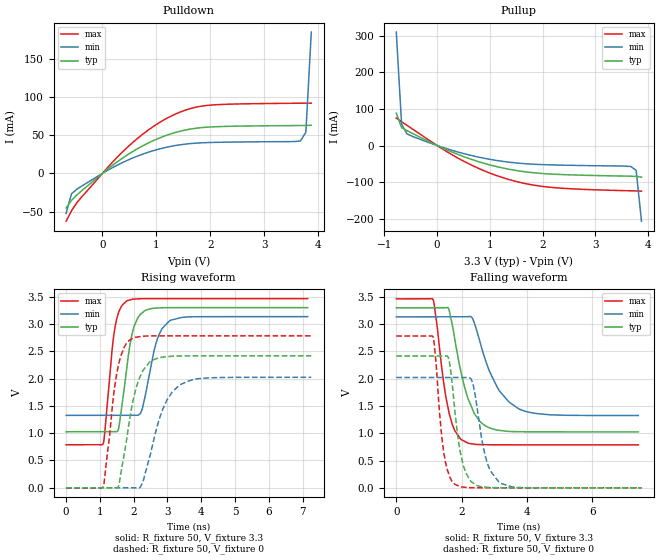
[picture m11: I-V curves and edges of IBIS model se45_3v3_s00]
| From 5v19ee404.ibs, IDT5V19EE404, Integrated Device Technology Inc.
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[Model]   se45_3v3_s00
Model_type   Output
Polarity   Non-Inverting
|   typ   min   max
C_comp   2pF   1.5pF   2.5pF
Vmeas = 1.65V
Rref = 50
Cref = 0
Vref = 1.65V
|   typ   min   max
[Voltage range]   3.3V   3.135V   3.465V
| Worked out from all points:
|   slope of the pulldown table from 0 to 0.495 V, typ, clamps not added: 19.3 ohm
|   slope of the pullup table from 0 to 0.495 V, typ, clamps not added: 16.5 ohm
|   rising waveform, R_fixture 50, V_fixture 3.3: 20-80 % time 317ps typ, 388ps min, 255ps max; typ from 1.03 V to 3.3 V
|   falling waveform, R_fixture 50, V_fixture 3.3: 20-80 % time 546ps typ, 767ps min, 379ps max; typ from 3.3 V to 1.03 V
|   rising waveform, R_fixture 50, V_fixture 0: 20-80 % time 444ps typ, 594ps min, 330ps max; typ from 0 V to 2.42 V
|   falling waveform, R_fixture 50, V_fixture 0: 20-80 % time 314ps typ, 381ps min, 254ps max; typ from 2.42 V to 0 V
[Pulldown]
|Voltage   I (typ)   I (min)   I (max)
|Note, modeling breaks down at 250mA and above.  This is well beyond the functional   |
|operating range of the device.  Should this scenario occur, catastrophic failure and   |
|possible damage to the device and/or board is of higher concern than the I-V curve   |
|behavior.  The IBIS checker will flag currents in excess of 10A with warnings.  Lines   |
|with currents in excess of 0.35 A have been commented out.  The points still remain|
|available to the user if the user desires to use them.   |
|-3.30000e+00   -6.87686e+01   -5.43171e+01   -9.32008e+01
|-3.19898e+00   -6.58203e+01   -5.20452e+01   -8.91014e+01
|-3.09796e+00   -6.28735e+01   -4.97746e+01   -8.50038e+01
|-2.99694e+00   -5.99283e+01   -4.75054e+01   -8.09081e+01
|-2.89592e+00   -5.69850e+01   -4.52379e+01   -7.68145e+01
|-2.79490e+00   -5.40436e+01   -4.29721e+01   -7.27232e+01
|-2.69388e+00   -5.11045e+01   -4.07082e+01   -6.86345e+01
|-2.59286e+00   -4.81679e+01   -3.84464e+01   -6.45487e+01
|-2.49184e+00   -4.52341e+01   -3.61871e+01   -6.04662e+01
|-2.39082e+00   -4.23034e+01   -3.39304e+01   -5.63874e+01
|-2.28980e+00   -3.93763e+01   -3.16768e+01   -5.23129e+01
|-2.18878e+00   -3.64533e+01   -2.94267e+01   -4.82433e+01
|-2.08776e+00   -3.35351e+01   -2.71807e+01   -4.41794e+01
|-1.98673e+00   -3.06226e+01   -2.49393e+01   -4.01225e+01
|-1.88571e+00   -2.77168e+01   -2.27035e+01   -3.60739e+01
|-1.78469e+00   -2.48192e+01   -2.04743e+01   -3.20355e+01
|-1.68367e+00   -2.19317e+01   -1.82533e+01   -2.80101e+01
|-1.58265e+00   -1.90571e+01   -1.60423e+01   -2.40013e+01
|-1.48163e+00   -1.61992e+01   -1.38443e+01   -2.00151e+01
|-1.38061e+00   -1.33643e+01   -1.16633e+01   -1.60610e+01
|-1.27959e+00   -1.05622e+01   -9.50583e+00   -1.21557e+01
|-1.17857e+00   -7.81131e+00   -7.38261e+00   -8.33341e+00
|-1.07755e+00   -5.14939e+00   -5.31366e+00   -4.68044e+00
|-9.76531e-01   -2.67462e+00   -3.34162e+00   -1.51483e+00
|-8.75510e-01   -7.31794e-01   -1.57851e+00   -1.44651e-01
|-7.74490e-01   -8.69816e-02   -3.68375e-01   -7.86452e-02
-673.5mV  -45.24mA   -52.43mA   -62.63mA
-572.4mV  -35.28mA   -26.51mA   -48.86mA
-471.4mV  -27.99mA   -20.59mA   -38.06mA
134.7mV   7.697mA    5.495mA    10.74mA
437.8mV   23.12mA    16.34mA    32.53mA
841.8mV   39.56mA    27.55mA    56.35mA
1.246V    51.27mA    35.11mA    74.04mA
1.65V     58.26mA    39.16mA    85.27mA
1.953V    60.57mA    40.35mA    89.06mA
3.67V     62.68mA    42.56mA    91.89mA
3.771V    62.76mA    53.73mA    91.95mA
3.872V    63.02mA    185mA      92.02mA
| 3.97347e+00   6.55596e-02   7.41798e-01   9.21553e-02
| 4.07449e+00   1.08647e-01   1.58880e+00   9.27153e-02
| 4.17551e+00   5.80299e-01   2.54532e+00   9.46081e-02
| 4.27653e+00   1.59953e+00   3.55180e+00   1.01817e-01
| 4.37755e+00   2.80777e+00   4.58590e+00   3.34477e-01
| 4.47857e+00   4.08831e+00   5.63734e+00   1.48889e+00
| 4.57959e+00   5.40528e+00   6.70059e+00   3.02324e+00
| 4.68061e+00   6.74390e+00   7.77238e+00   4.66566e+00
| 4.78163e+00   8.09679e+00   8.85061e+00   6.35541e+00
| 4.88265e+00   9.45977e+00   9.93391e+00   8.07133e+00
| 4.98367e+00   1.08302e+01   1.10213e+01   9.80380e+00
| 5.08469e+00   1.22065e+01   1.21119e+01   1.15477e+01
| 5.18571e+00   1.35874e+01   1.32054e+01   1.32998e+01
| 5.28673e+00   1.49721e+01   1.43012e+01   1.50583e+01
| 5.38776e+00   1.63599e+01   1.53991e+01   1.68219e+01
| 5.48878e+00   1.77503e+01   1.64987e+01   1.85895e+01
| 5.58980e+00   1.91430e+01   1.75998e+01   2.03604e+01
| 5.69082e+00   2.05377e+01   1.87024e+01   2.21342e+01
| 5.79184e+00   2.19342e+01   1.98062e+01   2.39105e+01
| 5.89286e+00   2.33322e+01   2.09111e+01   2.56888e+01
| 5.99388e+00   2.47315e+01   2.20170e+01   2.74690e+01
| 6.09490e+00   2.61321e+01   2.31238e+01   2.92508e+01
| 6.19592e+00   2.75338e+01   2.42314e+01   3.10341e+01
| 6.29694e+00   2.89366e+01   2.53398e+01   3.28186e+01
| 6.39796e+00   3.03402e+01   2.64489e+01   3.46043e+01
| 6.49898e+00   3.17447e+01   2.75587e+01   3.63909e+01
| 6.60000e+00   3.31499e+01   2.86691e+01   3.81786e+01
[Pullup]
|Voltage   I (typ)   I (min)   I (max)
|Note, modeling breaks down at 250mA and above.  This is well beyond the functional   |
|operating range of the device.  Should this scenario occur, catastrophic failure and   |
|possible damage to the device and/or board is of higher concern than the I-V curve   |
|behavior.  The IBIS checker will flag currents in excess of 10A with warnings.  Lines   |
|with currents in excess of 0.35 A have been commented out.  The points still remain|
|available to the user if the user desires to use them.   |
|-3.30000e+00   3.30685e+01   2.68041e+01   4.09731e+01
|-3.19898e+00   3.16649e+01   2.56956e+01   3.91868e+01
|-3.09796e+00   3.02620e+01   2.45879e+01   3.74012e+01
|-2.99694e+00   2.88598e+01   2.34808e+01   3.56164e+01
|-2.89592e+00   2.74585e+01   2.23744e+01   3.38325e+01
|-2.79490e+00   2.60582e+01   2.12689e+01   3.20497e+01
|-2.69388e+00   2.46589e+01   2.01643e+01   3.02679e+01
|-2.59286e+00   2.32607e+01   1.90607e+01   2.84873e+01
|-2.49184e+00   2.18638e+01   1.79583e+01   2.67082e+01
|-2.39082e+00   2.04684e+01   1.68571e+01   2.49306e+01
|-2.28980e+00   1.90746e+01   1.57574e+01   2.31549e+01
|-2.18878e+00   1.76827e+01   1.46593e+01   2.13812e+01
|-2.08776e+00   1.62931e+01   1.35631e+01   1.96100e+01
|-1.98673e+00   1.49060e+01   1.24691e+01   1.78417e+01
|-1.88571e+00   1.35221e+01   1.13777e+01   1.60769e+01
|-1.78469e+00   1.21418e+01   1.02894e+01   1.43164e+01
|-1.68367e+00   1.07662e+01   9.20489e+00   1.25612e+01
|-1.58265e+00   9.39630e+00   8.12499e+00   1.08130e+01
|-1.48163e+00   8.03397e+00   7.05098e+00   9.07412e+00
|-1.38061e+00   6.68178e+00   5.98471e+00   7.34826e+00
|-1.27959e+00   5.34400e+00   4.92891e+00   5.64201e+00
|-1.17857e+00   4.02815e+00   3.88819e+00   3.96831e+00
|-1.07755e+00   2.74939e+00   2.87074e+00   2.35829e+00
|-9.76531e-01   1.54478e+00   1.89336e+00   9.17339e-01
|-8.75510e-01   5.36288e-01   9.97523e-01   1.33296e-01
-774.5mV  88.48mA    310mA      75.29mA
-673.5mV  49mA       58.32mA    64.98mA
-572.4mV  40.75mA    31.76mA    55.15mA
-67.35mV  4.603mA    3.395mA    6.411mA
437.8mV   -26.87mA   -19.51mA   -37.82mA
841.8mV   -46.61mA   -33.39mA   -66.08mA
1.347V    -64.42mA   -45.25mA   -92.37mA
1.751V    -73.29mA   -50.54mA   -106.3mA
2.155V    -77.96mA   -52.94mA   -114.3mA
3.67V     -83.83mA   -57.37mA   -123.8mA
3.771V    -84.41mA   -67.8mA    -124.1mA
3.872V    -86.53mA   -207mA     -124.6mA
| 3.97347e+00   -9.23636e-02   -1.08741e+00   -1.26631e-01
| 4.07449e+00   -1.35075e-01   -2.71250e+00   -1.32720e-01
| 4.17551e+00   -7.98376e-01   -4.62912e+00   -1.42442e-01
| 4.27653e+00   -2.75140e+00   -6.66999e+00   -1.56925e-01
| 4.37755e+00   -5.22889e+00   -8.77650e+00   -4.29683e-01
| 4.47857e+00   -7.89161e+00   -1.09230e+01   -2.68260e+00
| 4.57959e+00   -1.06427e+01   -1.30961e+01   -6.10746e+00
| 4.68061e+00   -1.34446e+01   -1.52882e+01   -9.84047e+00
| 4.78163e+00   -1.62792e+01   -1.74945e+01   -1.36990e+01
| 4.88265e+00   -1.91366e+01   -1.97119e+01   -1.76242e+01
| 4.98367e+00   -2.20108e+01   -2.19380e+01   -2.15907e+01
| 5.08469e+00   -2.48978e+01   -2.41712e+01   -2.55849e+01
| 5.18571e+00   -2.77948e+01   -2.64103e+01   -2.95993e+01
| 5.28673e+00   -3.07000e+01   -2.86544e+01   -3.36287e+01
| 5.38776e+00   -3.36120e+01   -3.09027e+01   -3.76698e+01
| 5.48878e+00   -3.65296e+01   -3.31547e+01   -4.17205e+01
| 5.58980e+00   -3.94519e+01   -3.54100e+01   -4.57788e+01
| 5.69082e+00   -4.23784e+01   -3.76680e+01   -4.98436e+01
| 5.79184e+00   -4.53085e+01   -3.99286e+01   -5.39138e+01
| 5.89286e+00   -4.82418e+01   -4.21914e+01   -5.79887e+01
| 5.99388e+00   -5.11778e+01   -4.44562e+01   -6.20677e+01
| 6.09490e+00   -5.41163e+01   -4.67228e+01   -6.61502e+01
| 6.19592e+00   -5.70570e+01   -4.89910e+01   -7.02359e+01
| 6.29694e+00   -5.99998e+01   -5.12608e+01   -7.43243e+01
| 6.39796e+00   -6.29443e+01   -5.35319e+01   -7.84152e+01
| 6.49898e+00   -6.58905e+01   -5.58042e+01   -8.25083e+01
| 6.60000e+00   -6.88383e+01   -5.80778e+01   -8.66035e+01
[Ramp]
|   typ   min   max
dV/dt_r   1.364/0.316n   1.085/0.387n   1.606/0.254n
dV/dt_f   1.368/0.546n   1.089/0.767n   1.608/0.379n
R_load =   50.0000
[Rising Waveform]
R_fixture = 50
V_fixture = 3.3   |Vcc_typ
V_fixture_min = 3.135 |Vcc_min
V_fixture_max = 3.465 |Vcc_max
C_fixture = 0.0p
| Time   typ   min   max
0s        1.026V     1.326V     788.2mV
1.107ns   1.026V     1.326V     824.6mV
1.456ns   1.025V     1.326V     2.969V
1.568ns   1.124V     1.326V     3.235V
1.793ns   2.187V     1.326V     3.421V
1.976ns   2.875V     1.326V     3.455V
2.192ns   3.175V     1.354V     3.463V
2.687ns   3.293V     2.696V     3.465V
3.094ns   3.299V     3.069V     3.465V
7.151ns   3.3V       3.135V     3.465V
[Falling Waveform]
R_fixture = 50
V_fixture = 3.3   |Vcc_typ
V_fixture_min = 3.135 |Vcc_min
V_fixture_max = 3.465 |Vcc_max
C_fixture = 0.0p
| Time   typ   min   max
0s        3.3V       3.135V     3.465V
1.13ns    3.3V       3.135V     3.45V
1.437ns   3.3V       3.135V     1.982V
1.61ns    3.274V     3.135V     1.391V
1.973ns   2.142V     3.135V     889.6mV
2.335ns   1.435V     3.107V     804.7mV
2.567ns   1.215V     2.659V     792.4mV
3.149ns   1.053V     1.78V      788.7mV
3.75ns    1.029V     1.446V     788.4mV
7.403ns   1.026V     1.326V     788.3mV
[Rising Waveform]
R_fixture = 50
V_fixture = 0
C_fixture = 0.0p
| Time   typ   min   max
0s        124.7nV    139.7nV    109.3nV
1.113ns   -530.1nV   139.7nV    34.06mV
1.498ns   -1.108mV   94.01nV    2.089V
1.582ns   111.2mV    -213.9nV   2.327V
1.901ns   1.329V     40.44uV    2.715V
2.196ns   2.044V     8.88mV     2.769V
2.473ns   2.301V     558.7mV    2.781V
2.872ns   2.395V     1.453V     2.783V
3.356ns   2.414V     1.881V     2.783V
7.26ns    2.417V     2.024V     2.783V
[Falling Waveform]
R_fixture = 50
V_fixture = 0
C_fixture = 0.0p
| Time   typ   min   max
0s        2.417V     2.024V     2.783V
1.115ns   2.417V     2.024V     2.78V
1.456ns   2.417V     2.024V     633.5mV
1.613ns   2.347V     2.024V     239.3mV
1.793ns   1.402V     2.024V     64.87mV
2.162ns   237.9mV    2.024V     4.747mV
2.342ns   92.39mV    1.918V     1.759mV
2.766ns   9.04mV     489.7mV    288.2uV
3.154ns   1.387mV    92.08mV    185.3uV
7.5ns     79.55uV    144.4uV    43.91uV
